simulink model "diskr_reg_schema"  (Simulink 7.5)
settings: Solver=ode45  StartTime=0.0  StopTime=50  RelTol=1e-3
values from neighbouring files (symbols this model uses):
  den = [5 6 1]    [example_3_6_3_podklad.m]    (also in lmf2rat.m = mat2pol(den); lmf2tf.m = pol2mat(mat2pol(den).'))
  Grcit = pol2mat(reverse(Ccit_DpOK))    [example_3_6_3_podklad.m]
  Grjm = pol2mat(reverse(Cjmn_DpOK))    [example_3_6_3_podklad.m]
  num = 1    [example_3_6_3_podklad.m]    (also in lmf2rat.m = mat2pol(num); lmf2tf.m = pol2mat(mat2pol(num).'))
  T = 5    [example_3_6_3_podklad.m]    (also in axxab.m = T(:, select); bhf.m = eye(sumbsizes); charact.m = [[T(1:n,:) newT]; [zeros(order*n,n) T]]; h2.m = [     D11      D12*Xo-N12*Yo)

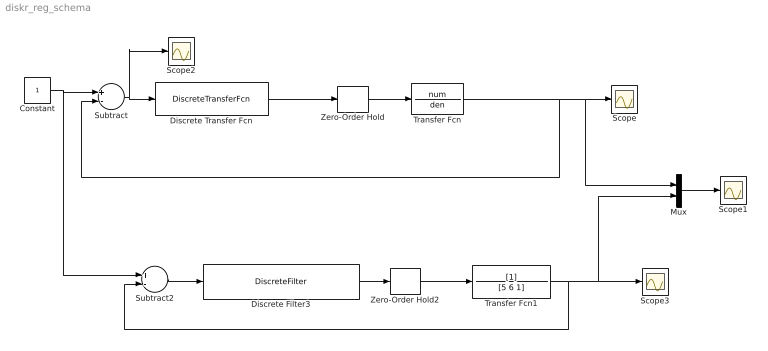
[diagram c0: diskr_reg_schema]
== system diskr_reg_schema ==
  Constant : Constant
  Discrete Transfer Fcn : DiscreteTransferFcn  Numerator=Grcit  Denominator=Grjm  SampleTime=T
  Discrete Filter3 : DiscreteFilter  Numerator=[1.5926 -0.59659 0.0039815]  Denominator=[1 -0.8629 -0.1371]  SampleTime=5
  Mux : Mux  Inputs=2
  Scope{,1..3} (4 alike) : Scope
  Subtract : Sum  Inputs=+-
  Subtract2 : Sum  Inputs=+-
  Transfer Fcn : TransferFcn  Numerator=num  Denominator=den
  Transfer Fcn1 : TransferFcn  Denominator=[5 6 1]
  Zero-Order Hold : ZeroOrderHold  SampleTime=T
  Zero-Order Hold2 : ZeroOrderHold  SampleTime=5
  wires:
  Constant/1 -> Subtract/1, Subtract2/1
  Subtract/1 -> Discrete Transfer Fcn/1, Scope2/1
  Discrete Transfer Fcn/1 -> Zero-Order Hold/1
  Transfer Fcn/1 -> Subtract/2, Scope/1, Mux/1
  Zero-Order Hold/1 -> Transfer Fcn/1
  Subtract2/1 -> Discrete Filter3/1
  Discrete Filter3/1 -> Zero-Order Hold2/1
  Transfer Fcn1/1 -> Subtract2/2, Scope3/1, Mux/2
  Zero-Order Hold2/1 -> Transfer Fcn1/1
  Mux/1 -> Scope1/1
